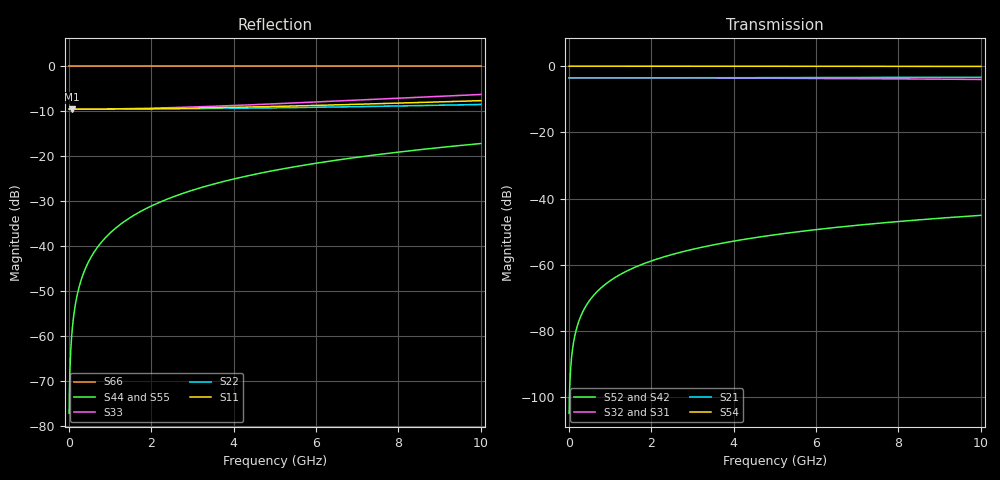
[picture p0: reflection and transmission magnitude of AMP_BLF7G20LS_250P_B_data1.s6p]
! Created Thu Oct 28 10:55:25 2010
# ghz S ma R 50
! 6 Port Network Data from SP1.SP block
! freq  magS11  angS11  magS12  angS12  magS13  angS13  magS14  angS14
!  magS15  angS15  magS16  angS16
!  magS21  angS21  magS22  angS22
!  magS23  angS23  magS24  angS24  magS25  angS25  magS26  angS26
!  magS31  angS31  magS32  angS32  magS33  angS33  magS34  angS34
!  magS35  angS35  magS36  angS36
!  magS41  angS41  magS42  angS42
!  magS43  angS43  magS44  angS44  magS45  angS45  magS46  angS46
!  magS51  angS51  magS52  angS52  magS53  angS53  magS54  angS54
!  magS55  angS55  magS56  angS56
!  magS61  angS61  magS62  angS62
!  magS63  angS63  magS64  angS64  magS65  angS65  magS66  angS66
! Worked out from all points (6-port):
!   1000 points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, 10 MHz to 10 GHz, reference 50 ohm
!   strongest paths, dB at 10 MHz, 2.51 GHz, 5.01 GHz, 7.51 GHz, 10 GHz:
!     S54: 0.0, 0.0, 0.0, 0.0, -0.1
!     S21: -3.5, -3.5, -3.5, -3.4, -3.4
!     S32: -3.5, -3.6, -3.7, -3.8, -4.0
!     S31: -3.5, -3.6, -3.7, -4.0, -4.4
!     S52: -104.9, -56.9, -50.9, -47.5, -45.1
!     S42: -104.9, -56.9, -50.9, -47.5, -45.1
!   lowest |S11| = -9.5 dB at 80 MHz (marker M1), VSWR 2.00, Z = 25 + j0.182 ohm
!   |S11| at or under -10 dB: nowhere
